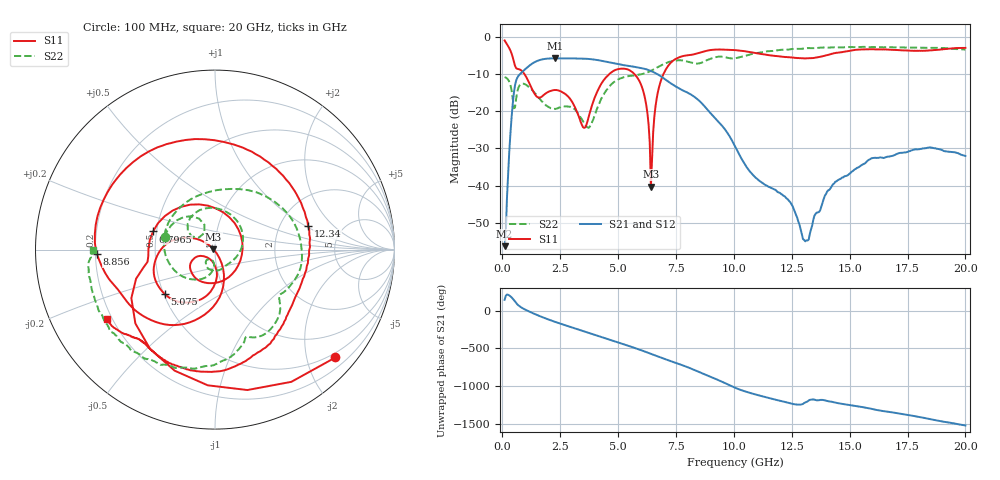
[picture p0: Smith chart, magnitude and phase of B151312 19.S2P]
!  2-Port S-parameters saved by WinCal
! VAR MeasName=S-Parameters (CALIBRATED_DATA) read from VNA (N5244A)
! VAR MeasDate=12/8/2015 5:44:56 PM
! VAR NAME=B151312 19
! VAR FILENAME=B151312 19.S2P
! VAR DATE=12/8/2015 5:44:56 PM
! VAR PHYS_PORTS=1,2
# Hz S DB R 50
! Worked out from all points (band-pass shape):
!   401 points, 100 MHz to 20 GHz, reference 50 ohm
!   highest |S21| = -5.74 dB at 2.289 GHz (marker M1); lowest = -56.3 dB at 100 MHz (marker M2)
!   |S21| within 3 dB of the highest: 974.3 MHz to 6.249 GHz (5.275 GHz wide, 146 % of centre)
!   lowest |S11| = -40.2 dB at 6.418 GHz (marker M3), VSWR 1.02, Z = 49.1 + j0.258 ohm
!   |S11| at or under -10 dB: 958.8 MHz to 4.617 GHz (3.658 GHz wide, 131 % of centre); 5.712 GHz to 6.958 GHz (1.246 GHz wide, 19.7 % of centre)
!   |S22| runs from -24.4 to -2.6 dB; largest |S21 - S12| = 0.0016
!   S11 on the Smith chart (normalised r, x): 100 MHz: 0.40, -2.56; 796.5 MHz: 0.48, +0.11; 5.075 GHz: 0.51, -0.29; 8.856 GHz: 0.21, -0.02; 12.34 GHz: 2.87, +1.06; 20 GHz: 0.18, -0.29
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1e8  -0.91 -41.9  -56.31 144.9  -56.66 145.7  -10.76 165.9
4.4825e8  -5.37 -149.9  -18.14 161.6  -18.14 161.5  -16.47 113.0
7.965e8  -8.87 163.7  -9.78 48.7  -9.78 48.7  -12.69 119.7
1.1945e9  -12.79 88.6  -7.57 -15.2  -7.57 -15.2  -13.68 58.8
1.64225e9  -16.25 -23.2  -6.13 -74.6  -6.13 -74.6  -16.81 -0.0
2.289e9  -14.25 -115.8  -5.74 -148.7  -5.74 -148.7  -19.37 -55.1
3.43325e9  -23.56 -142.9  -5.79 95.7  -5.79 95.7  -22.11 -129.0
4.22925e9  -13.08 -94.2  -6.30 15.2  -6.30 15.1  -17.24 -101.0
5.075e9  -8.55 -138.4  -7.34 -69.0  -7.34 -69.0  -11.18 -172.2
5.9705e9  -12.49 166.9  -8.31 -161.4  -8.32 -161.6  -10.03 107.6
6.41825e9  -40.24 164.3  -9.12 147.6  -9.12 147.7  -9.11 74.7
6.7665e9  -13.53 -77.5  -10.24 107.1  -10.24 107.1  -7.92 50.2
7.61225e9  -5.52 -132.2  -13.75 14.3  -13.71 14.2  -6.24 -6.6
8.856e9  -3.65 -177.7  -19.52 -140.6  -19.48 -140.9  -6.17 -42.2
1.005e10  -3.51 133.0  -29.40 57.0  -29.45 56.8  -5.71 -70.8
1.11445e10  -4.51 79.9  -38.87 -49.7  -38.92 -49.9  -4.17 -85.6
1.23385e10  -5.43 14.2  -43.74 -142.2  -43.79 -141.0  -3.36 -104.4
1.308475e10  -5.73 -20.6  -55.00 -138.2  -55.07 -139.2  -3.01 -114.7
1.338325e10  -5.67 -31.2  -50.73 -99.8  -50.59 -99.1  -3.00 -117.6
1.437825e10  -4.31 -61.0  -38.98 -140.1  -38.91 -139.4  -2.72 -129.6
1.67165e10  -3.40 -114.4  -32.20 95.0  -32.03 95.1  -2.72 -152.3
2e10  -2.91 -147.1  -32.02 -84.0  -32.09 -85.3  -3.37 180.0
